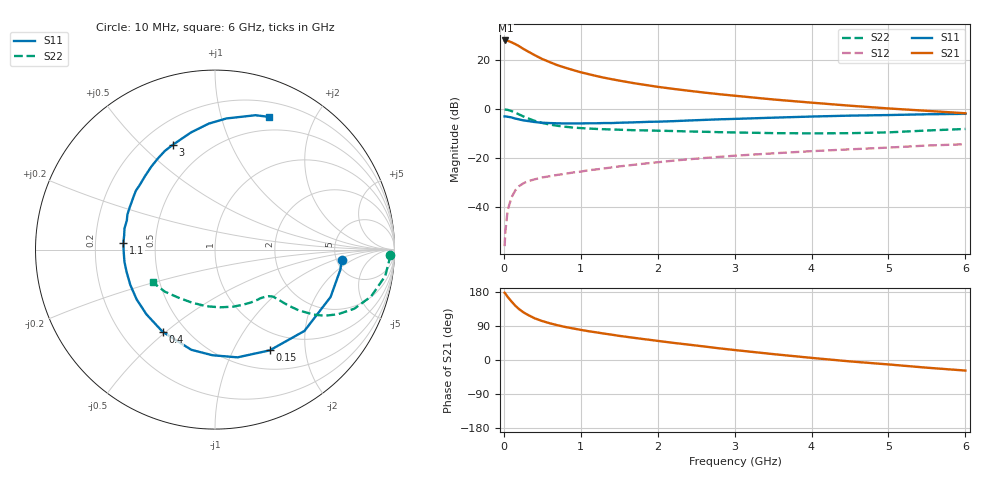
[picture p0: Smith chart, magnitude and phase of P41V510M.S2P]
! SIEMENS Small Signal Semiconductors
! BFP182
! Si NPN RF Bipolar Junction Transistor in SOT143
! VCE = 1.5 V  IC = 10 mA
! Common Emitter S-Parameters:  March  1996
# GHz  S  MA  R  50
!  f  S11  S21  S12  S22
! GHz  MAG  ANG  MAG  ANG  MAG  ANG  MAG  ANG
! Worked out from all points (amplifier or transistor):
!   36 points, 10 MHz to 6 GHz, reference 50 ohm
!   highest |S21| = 28.0 dB at 20 MHz (marker M1)
!   |S21| within 3 dB of that: start of sweep to 231.6 MHz
!   unconditionally stable (mu >= 1): 1.041 GHz to 5.43 GHz
!   at 250 MHz: K = 0.35, MSG = 27.5 dB, |S12| = -30.4 dB
!   at 1.4 GHz: K = 1.12, MAG = 15.8 dB, |S12| = -23.8 dB
!   at 6 GHz: K = 0.95, MSG = 6.3 dB, |S12| = -14.4 dB
!   S11 on the Smith chart (normalised r, x): 10 MHz: 5.57, -1.24; 150 MHz: 0.74, -1.41; 400 MHz: 0.38, -0.49; 1.1 GHz: 0.32, +0.03; 3 GHz: 0.32, +0.62; 6 GHz: 0.35, +1.42
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0.01  0.7081 -4.5  24.83 177.5  0.0016 86.2  0.9772 -1.7
0.02  0.7076 -9.0  25 175.0  0.0032 84.6  0.9728 -3.5
0.05  0.696 -22.3  24.67 166.5  0.0087 79.6  0.9599 -8.8
0.1  0.6735 -42.3  22.88 154.3  0.0158 69.4  0.9081 -16.7
0.15  0.6388 -61.5  21.07 143.1  0.0221 61.9  0.843 -23.0
0.2  0.6133 -78.2  19.03 133.9  0.0269 56.7  0.7731 -27.8
0.25  0.5887 -91.4  16.96 126.5  0.0303 52.2  0.7117 -31.2
0.3  0.5736 -103.3  15.33 120.4  0.0332 49.4  0.6578 -33.4
0.4  0.5431 -122.5  12.56 110.1  0.0369 45.7  0.5748 -36.0
0.5  0.5253 -136.7  10.45 102.7  0.0403 43.5  0.5189 -37.2
0.6  0.5173 -147.5  9.002 96.8  0.0428 43.2  0.4817 -37.8
0.7  0.5113 -157.3  7.796 91.6  0.0455 42.4  0.4545 -38.2
0.9  0.5091 -172.3  6.235 83.3  0.0509 43.4  0.419 -38.9
1.1  0.512 176.0  5.152 76.0  0.0565 44.0  0.4004 -40.5
1.5  0.5257 158.2  3.797 63.7  0.0677 44.2  0.3787 -44.6
1.8  0.5422 146.5  3.166 55.6  0.0763 44.2  0.368 -48.9
2.2  0.5654 133.6  2.579 45.3  0.0884 42.5  0.3564 -55.7
3  0.6292 112.0  1.868 26.3  0.1117 37.8  0.3332 -72.7
3.5  0.6663 101.6  1.568 15.6  0.1248 34.1  0.3226 -85.3
4.5  0.7336 85.0  1.169 -3.7  0.1508 26.7  0.3218 -113.0
5.5  0.7816 73.3  0.918 -20.3  0.1801 19.1  0.3648 -140.0
6  0.7979 68.0  0.82 -27.9  0.1916 14.3  0.3923 -152.5
